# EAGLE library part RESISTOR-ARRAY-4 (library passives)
Chip resistor array Example part: 1K array Digikey Y7102CT-ND
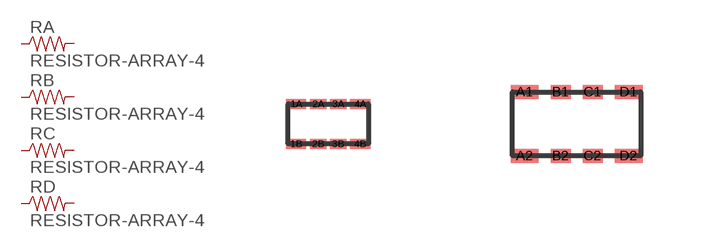
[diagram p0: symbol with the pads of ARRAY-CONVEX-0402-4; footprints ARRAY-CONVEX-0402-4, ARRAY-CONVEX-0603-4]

Designator prefix R; gates A=RESISTOR B=RESISTOR C=RESISTOR D=RESISTOR

## RESISTOR-ARRAY-40804  [ARRAY-CONVEX-0402-4]
1A  A:1  pas
1B  A:2  pas
2A  B:1  pas
2B  B:2  pas
3A  C:1  pas
3B  C:2  pas
4A  D:1  pas
4B  D:2  pas

## RESISTOR-ARRAY-41206  [ARRAY-CONVEX-0603-4]
A1  A:1  pas
A2  A:2  pas
B1  B:1  pas
B2  B:2  pas
C1  C:1  pas
C2  C:2  pas
D1  D:1  pas
D2  D:2  pas

## Footprint ARRAY-CONVEX-0402-4 (pad centres in mm)
Chip Resistor Array - 0804 package - 4x0402 Drawn from https://industrial.panasonic.com/cdbs/www-data/pdf/AOC0000/AOC0000C14.pdf From DigiKey part Y7102CT-ND
smd 0.5 x 0.25: 1A -0.8,0.5; 1B -0.8,-0.5; 4A 0.8,0.5; 4B 0.8,-0.5
smd 0.4 x 0.25: 2A -0.25,0.5; 2B -0.25,-0.5; 3A 0.25,0.5; 3B 0.25,-0.5

## Footprint ARRAY-CONVEX-0603-4 (pad centres in mm)
Chip Resistor Array - 1206 - 4x0603 Drawn from https://industrial.panasonic.com/cdbs/www-data/pdf/AOC0000/AOC0000C14.pdf Digikey part Y9102CT-ND
smd 0.7 x 0.35: A1 -1.3,0.8; A2 -1.3,-0.8; D1 1.3,0.8; D2 1.3,-0.8
smd 0.5 x 0.35: B1 -0.4,0.8; B2 -0.4,-0.8; C1 0.4,0.8; C2 0.4,-0.8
